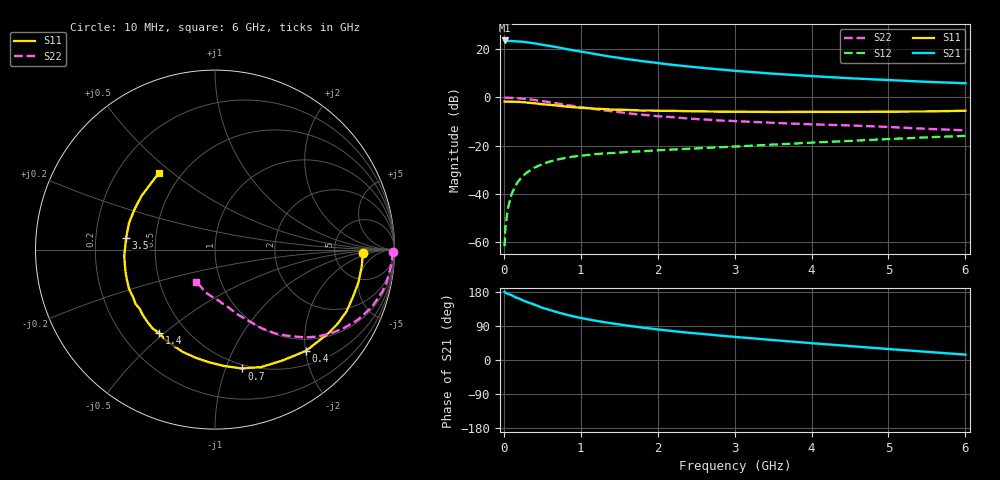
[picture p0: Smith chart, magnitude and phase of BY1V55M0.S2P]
! SIEMENS Small Signal Semiconductors
! BFY420
! Si NPN RF SIEGET Grounded Emitter Transistor in MICRO-X
! VCE = 1.5 V  IC = 5 mA
! Common Emitter S-Parameters:  October  1996
# GHz  S  MA  R  50
!  f  S11  S21  S12  S22
! GHz  MAG  ANG  MAG  ANG  MAG  ANG  MAG  ANG
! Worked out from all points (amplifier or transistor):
!   36 points, 10 MHz to 6 GHz, reference 50 ohm
!   highest |S21| = 23.8 dB at 10 MHz (marker M1)
!   |S21| within 3 dB of that: start of sweep to 722.3 MHz
!   unconditionally stable (mu >= 1): 3.117 GHz to end of sweep
!   at 250 MHz: K = 0.11, MSG = 27.9 dB, |S12| = -32.7 dB
!   at 1.4 GHz: K = 0.54, MSG = 20.1 dB, |S12| = -23.2 dB
!   at 6 GHz: K = 1.15, MAG = 8.6 dB, |S12| = -16.0 dB
!   S11 on the Smith chart (normalised r, x): 10 MHz: 10, -1; 400 MHz: 0.76, -2.01; 700 MHz: 0.46, -1.14; 1.4 GHz: 0.35, -0.48; 3.5 GHz: 0.34, +0.06; 6 GHz: 0.38, +0.45
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0.01  0.8267 -1.5  15.43 180.0  0.0008 96.7  0.9904 -0.7
0.02  0.8234 -2.7  15.34 177.6  0.0019 78.0  0.9917 -1.3
0.05  0.8229 -6.4  15.06 174.7  0.0047 85.4  0.9877 -3.4
0.1  0.8198 -12.8  15.03 171.1  0.0096 84.4  0.9806 -7.0
0.15  0.8126 -18.9  14.79 165.6  0.0146 79.1  0.9731 -10.5
0.2  0.8095 -25.2  14.68 162.0  0.019 77.6  0.9627 -13.8
0.25  0.7989 -31.0  14.44 157.3  0.0233 73.3  0.9453 -17.1
0.3  0.785 -36.5  14.1 153.1  0.0275 71.3  0.9292 -20.3
0.4  0.7584 -48.1  13.42 145.9  0.0347 65.7  0.8868 -26.2
0.5  0.723 -58.8  12.55 137.9  0.0408 60.7  0.8402 -31.4
0.6  0.7033 -68.6  11.85 131.8  0.0467 56.4  0.7942 -36.1
0.7  0.6783 -77.4  11.1 125.8  0.0512 52.9  0.749 -40.3
0.9  0.6285 -93.1  9.631 115.3  0.0588 47.1  0.6661 -46.8
1.1  0.5982 -107.3  8.529 107.0  0.0637 43.1  0.5971 -52.5
1.4  0.5601 -123.7  7.024 96.8  0.0694 38.9  0.5179 -58.7
1.8  0.5338 -141.7  5.719 85.6  0.0758 35.8  0.4384 -64.9
2.2  0.5263 -155.7  4.774 76.3  0.0825 34.1  0.3883 -70.1
2.8  0.5081 -171.9  3.848 64.6  0.0918 32.8  0.3319 -76.7
3.5  0.4994 172.7  3.134 52.6  0.1045 30.9  0.2965 -83.4
4.5  0.5013 153.3  2.517 36.7  0.1248 26.9  0.2618 -94.3
5.5  0.5123 134.6  2.12 21.6  0.1478 21.2  0.2222 -110.4
6  0.5293 126.4  1.984 14.1  0.1591 17.8  0.2066 -120.6
